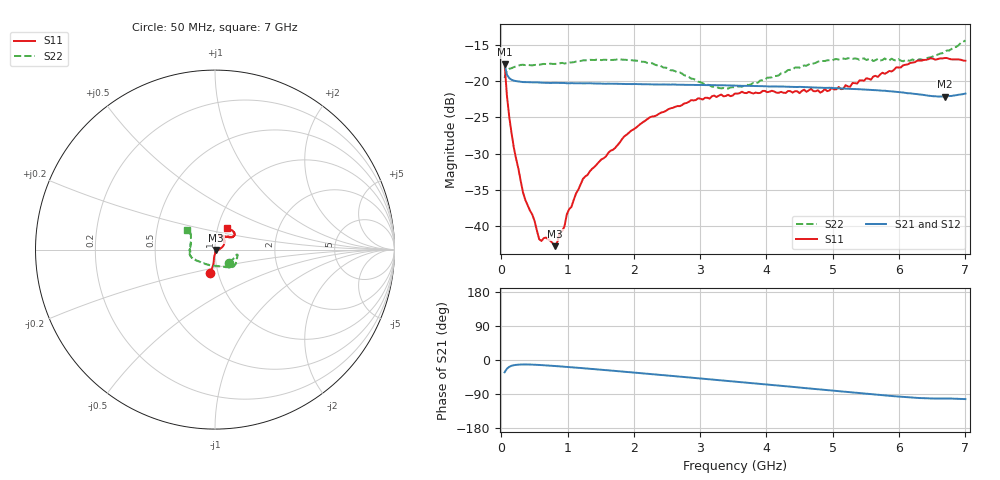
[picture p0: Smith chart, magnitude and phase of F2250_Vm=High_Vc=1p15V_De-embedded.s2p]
! Integrated Device Technology
! Corporate Headquarters
! 6024 Silver Creek Valley Road
! San Jose, CA 95138  USA
! Phone:  1-408-284-8200
! Toll Free:  1-800-223-1366
! Webpage:  http://www.idt.com/
! Timing and RF Division
! 515 Groton Road, Suite 102
! Westford, MA 01886-6024
! Device:  F2250
! Description: Voltage Variable RF Attenuator
! Frequency:  50.0 -  6000.00 MHz
! Package:  3x3 mm Thin QFN Plastic Package: 16 pin
! Ports:  2 RF, 3 DC
!  Pin  1  = GND
!  Pin  2  = NC
!  Pin  3  = RF1  = Port 1
!  Pin  4  = NC
!  Pin  5  = GND
!  Pin  6  = GND
!  Pin  7  = GND
!  Pin  8  = GND
!  Pin  9  = NC
!  Pin 10  = RF2  = Port 2
!  Pin 11  = NC
!  Pin 12  = GND
!  Pin 13  = GND
!  Pin 14  = VCNTRL
!  Pin 15  = VDD
!  Pin 16  = VMODE
! Vcntrl:  1.150 Volts
! Vmode:  +3.300 Volts
! Vdd:  +3.30  Volts
! Current:  1.330 mA
! Data:  The device was measured on a the F2250 evaluation board which has
!  individual transmission lines to the RF pins.  Data was collected
!  using a calibrated network analyzer.  The evaluation board was
!  de-embedded using a TRL calibration technique.
!  The reference plane is the edge of the package pin.
! Misc:  SN 10
!  Action Tracker AT0258
! Date Measured:  2014-11-26
! Date:  2015-10-15  MJV
! Note:
!  Integrated Device Technology supplies this data as a sample of measured
!  data at the package pin for this product.  Your particular data for this
!  product may vary.
!  Data was taken at 25 degrees C.
!  Integrated Device Technology reserves the right to change this data at anytime.
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# GHz S dB R 50
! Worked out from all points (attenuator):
!   201 points, 50 MHz to 7 GHz, reference 50 ohm
!   highest |S21| = -17.69 dB at 50 MHz (marker M1); lowest = -22.1 dB at 6.687 GHz (marker M2)
!   lowest |S11| = -42.7 dB at 814.5 MHz (marker M3), VSWR 1.01, Z = 50.7 - j0.283 ohm
!   |S11| at or under -10 dB: start of sweep to end of sweep
!   |S22| runs from -21.0 to -14.4 dB; largest |S21 - S12| = 0.0003
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0.05  -17.62 -101.1  -17.69 -32.5  -17.69 -32.5  -19.55 -43.8
0.08475  -21.98 -96.0  -19.11 -23.0  -19.10 -22.9  -18.49 -22.0
0.15425  -27.15 -97.0  -19.81 -15.4  -19.81 -15.4  -18.22 -13.6
0.328  -35.35 -87.1  -20.13 -11.7  -20.11 -11.7  -17.75 -12.8
0.50175  -39.25 -71.6  -20.17 -12.5  -20.17 -12.5  -17.78 -16.1
0.57125  -41.77 -58.3  -20.20 -13.1  -20.20 -13.1  -17.74 -17.6
0.6755  -41.55 -51.4  -20.23 -14.2  -20.23 -14.2  -17.65 -19.7
0.8145  -42.74 -22.5  -20.24 -15.9  -20.24 -15.9  -17.63 -23.5
0.884  -40.86 -19.1  -20.25 -16.8  -20.25 -16.8  -17.54 -25.7
0.9535  -40.00 -24.7  -20.26 -17.7  -20.27 -17.7  -17.57 -27.0
0.98825  -38.36 -20.8  -20.29 -18.2  -20.28 -18.2  -17.52 -27.7
1.2315  -33.48 -1.3  -20.31 -21.6  -20.30 -21.6  -17.14 -32.6
1.857  -27.59 18.4  -20.39 -31.0  -20.39 -31.0  -17.04 -42.2
2.37825  -24.50 31.7  -20.48 -38.9  -20.46 -39.0  -17.78 -50.9
3.1775  -22.08 53.9  -20.56 -51.5  -20.57 -51.5  -20.77 -82.6
3.525  -21.70 64.4  -20.62 -57.1  -20.62 -57.1  -20.83 -106.7
4.7065  -21.38 68.4  -20.87 -76.1  -20.87 -76.1  -17.57 -158.0
5.15825  -21.06 51.9  -21.03 -83.4  -21.01 -83.4  -16.89 -167.0
5.85325  -18.60 36.8  -21.39 -94.5  -21.39 -94.6  -17.13 177.7
6.3745  -17.08 38.4  -21.91 -101.0  -21.92 -101.0  -17.08 159.8
6.68725  -16.82 45.9  -22.14 -101.8  -22.13 -102.0  -15.96 147.9
7  -17.20 61.9  -21.71 -103.2  -21.72 -103.3  -14.40 144.4
